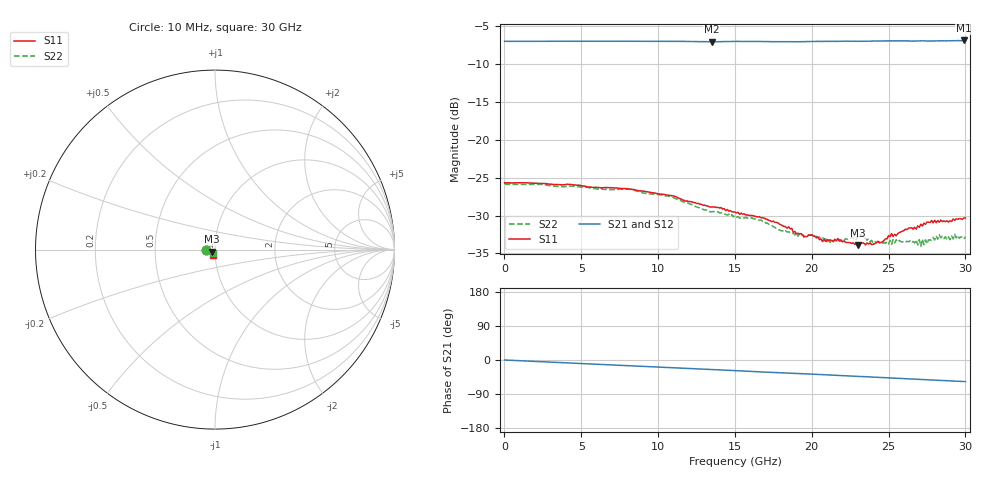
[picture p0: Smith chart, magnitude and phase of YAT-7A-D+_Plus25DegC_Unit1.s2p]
!Keysight Technologies,N5244A,MY52442000,A.10.40.14
!Model Number: YAT-7A-D+
!Date: Wednesday, October 26, 2016 14:48:10
!Correction: S11(Full 2 Port(1,2))
!S21(Full 2 Port(1,2))
!S12(Full 2 Port(1,2))
!S22(Full 2 Port(1,2))
!S2P File: Measurements: S11, S21, S12, S22:
# Hz S  dB  R 50
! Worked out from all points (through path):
!   309 points, 10 MHz to 30 GHz, reference 50 ohm
!   highest |S21| = -6.89 dB at 29.9 GHz (marker M1); lowest = -7.1 dB at 13.5 GHz (marker M2)
!   group delay of S21, straight-line fit = 5.26 ps
!   lowest |S11| = -33.9 dB at 23 GHz (marker M3), VSWR 1.04, Z = 48.3 - j1.04 ohm
!   |S11| at or under -10 dB: start of sweep to end of sweep
!   |S22| runs from -34.0 to -25.8 dB; largest |S21 - S12| = 0.0028
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1e7  -25.67 -179.9  -7.01 0.0  -7.00 0.0  -25.86 -179.8
5.1e9  -26.08 176.2  -7.00 -9.4  -7.00 -9.4  -26.23 175.1
1.01e10  -27.18 173.2  -7.00 -19.0  -6.99 -19.0  -27.26 168.9
1.35e10  -28.86 173.9  -7.07 -25.3  -7.06 -25.3  -29.49 170.5
1.51e10  -29.65 178.4  -7.01 -28.2  -7.01 -28.1  -30.21 172.7
1.67e10  -30.28 178.4  -7.03 -31.4  -7.02 -31.4  -30.58 174.1
1.91e10  -32.32 -172.3  -7.05 -35.7  -7.06 -35.6  -32.73 -176.4
2.01e10  -32.73 -168.8  -7.02 -37.5  -7.01 -37.4  -32.62 -173.3
2.12e10  -33.22 -157.9  -7.00 -39.7  -7.00 -39.5  -33.57 -165.3
2.3e10  -33.91 -147.6  -7.01 -43.2  -7.00 -43.1  -32.71 -156.8
2.4e10  -33.79 -139.3  -6.96 -45.0  -6.99 -45.0  -33.63 -153.6
2.51e10  -32.77 -128.4  -6.95 -47.3  -6.93 -47.3  -33.28 -153.5
2.68e10  -31.79 -123.2  -6.97 -50.8  -6.95 -50.7  -33.21 -138.8
2.69e10  -31.36 -122.6  -6.95 -51.1  -6.94 -50.8  -33.87 -136.7
2.7e10  -31.56 -122.4  -6.96 -51.2  -6.96 -51.1  -33.17 -138.0
2.71e10  -31.15 -121.7  -6.95 -51.5  -6.95 -51.3  -34.04 -137.0
2.72e10  -31.38 -122.9  -6.94 -51.5  -6.96 -51.6  -33.12 -136.0
2.73e10  -31.01 -121.2  -6.95 -51.7  -6.96 -51.8  -33.83 -139.1
2.74e10  -31.15 -123.0  -6.95 -51.8  -6.97 -52.1  -33.19 -134.6
2.83e10  -30.88 -120.0  -6.95 -53.7  -6.93 -53.6  -32.54 -137.3
2.99e10  -30.32 -116.2  -6.89 -56.8  -6.92 -56.9  -33.10 -123.3
3e10  -30.30 -114.0  -6.91 -57.0  -6.88 -57.0  -32.80 -126.2
